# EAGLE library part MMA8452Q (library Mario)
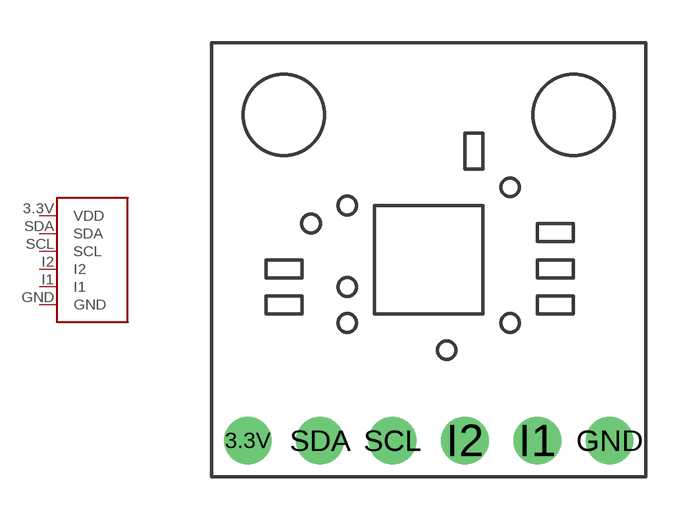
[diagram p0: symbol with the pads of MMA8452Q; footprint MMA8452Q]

Designator prefix -

## MMA8452Q  [MMA8452Q]
3.3V  VDD
GND  GND
I1  I1
I2  I2
SCL  SCL
SDA  SDA

## Footprint MMA8452Q (pad centres in mm)
drill 0.6 pad 1.676: 3.3V -6.35,-6.35; GND 6.35,-6.35; I1 3.81,-6.35; I2 1.27,-6.35; SCL -1.27,-6.35; SDA -3.81,-6.35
